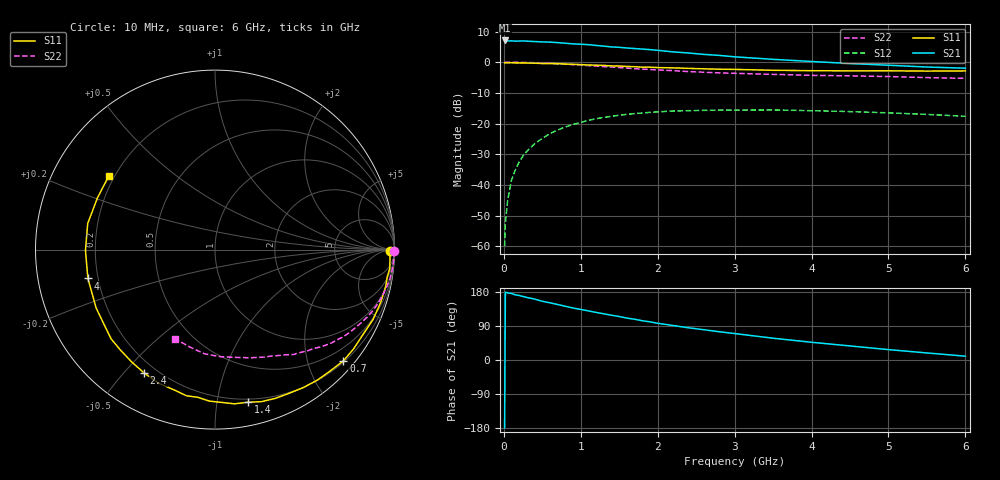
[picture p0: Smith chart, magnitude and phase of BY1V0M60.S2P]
! SIEMENS Small Signal Semiconductors
! BFY420
! Si NPN RF SIEGET Grounded Emitter Transistor in MICRO-X
! VCE = 1 V  IC = 0.6 mA
! Common Emitter S-Parameters:  October  1996
# GHz  S  MA  R  50
!  f  S11  S21  S12  S22
! GHz  MAG  ANG  MAG  ANG  MAG  ANG  MAG  ANG
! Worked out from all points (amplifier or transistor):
!   36 points, 10 MHz to 6 GHz, reference 50 ohm
!   highest |S21| = 7.1 dB at 10 MHz (marker M1)
!   |S21| within 3 dB of that: start of sweep to 1.903 GHz
!   unconditionally stable (mu >= 1): 4.752 GHz to end of sweep
!   at 250 MHz: K = 0.04, MSG = 18.7 dB, |S12| = -30.5 dB
!   at 1.4 GHz: K = 0.22, MSG = 11.3 dB, |S12| = -17.6 dB
!   at 6 GHz: K = 1.38, MAG = 4.2 dB, |S12| = -17.6 dB
!   S11 on the Smith chart (normalised r, x): 10 MHz: 64, -25; 700 MHz: 0.22, -2.67; 1.4 GHz: 0.18, -1.22; 2.4 GHz: 0.15, -0.57; 4 GHz: 0.16, -0.11; 6 GHz: 0.18, +0.31
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0.01  0.9732 -0.6  2.261 -179.1  0.001 91.6  0.9999 -0.4
0.02  0.9743 -1.4  2.252 178.7  0.0024 88.4  0.9999 -0.7
0.05  0.9762 -3.0  2.214 177.1  0.0056 90.2  0.9976 -1.6
0.1  0.9795 -6.2  2.229 175.5  0.012 88.8  0.9969 -3.2
0.15  0.9713 -9.1  2.201 171.9  0.0175 84.2  0.996 -4.8
0.2  0.9731 -12.1  2.214 170.3  0.0237 82.6  0.9941 -6.3
0.25  0.9701 -15.0  2.222 167.5  0.0297 79.8  0.9903 -7.9
0.4  0.963 -23.8  2.17 160.8  0.0467 74.7  0.9784 -12.5
0.5  0.9506 -29.8  2.142 154.9  0.0572 70.6  0.9674 -15.5
0.7  0.9464 -40.9  2.086 146.4  0.0783 63.4  0.9414 -21.4
0.9  0.9238 -52.0  1.989 137.2  0.0967 56.0  0.9108 -26.6
1.1  0.9003 -63.1  1.931 129.5  0.1124 49.4  0.8793 -31.8
1.4  0.8699 -77.8  1.771 118.1  0.1311 40.2  0.8328 -38.6
1.8  0.8283 -96.7  1.635 103.6  0.1483 29.5  0.7717 -46.2
2.2  0.808 -112.7  1.472 91.0  0.1598 20.0  0.7287 -53.4
2.4  0.7928 -119.9  1.412 85.0  0.162 16.2  0.7025 -56.6
2.8  0.7688 -133.2  1.29 74.6  0.1653 8.9  0.6687 -62.6
3.5  0.7379 -153.8  1.113 57.5  0.1665 -1.2  0.6331 -72.2
4  0.7263 -167.2  1.027 46.8  0.1619 -7.3  0.6104 -79.5
4.5  0.7218 -179.7  0.951 37.1  0.1564 -12.7  0.5978 -87.0
5.5  0.7155 156.3  0.834 18.6  0.1408 -19.8  0.5606 -104.4
6  0.7205 145.1  0.798 10.1  0.1311 -21.3  0.5444 -114.3
